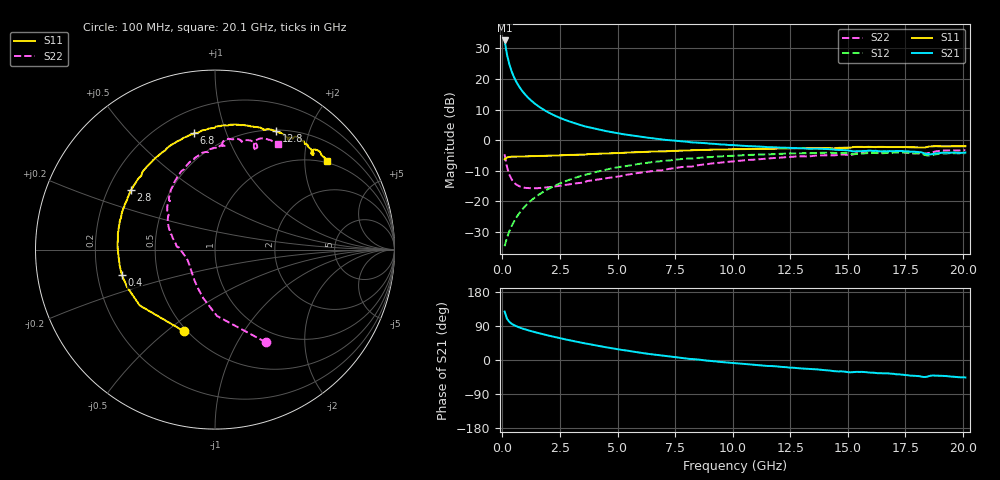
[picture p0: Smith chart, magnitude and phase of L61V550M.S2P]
!  Infineon Technologies AG
! BFR380L3 , PF131585-7, No.6, Th 09.10.01, soldered on pcb-board, measured with PP GSG850
!  Vce=1.5 V,  Ic=50.0 mA
! Common Emitter S-Parameters:  15. November 2001
#  GHz  S  MA  R  50
! f  S11  S21  S12  S22
! GHz  Mag  Ang  Mag  Ang  Mag  Ang  Mag  Ang
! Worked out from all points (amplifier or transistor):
!   201 points, 100 MHz to 20.1 GHz, reference 50 ohm
!   highest |S21| = 32.6 dB at 100 MHz (marker M1)
!   |S21| within 3 dB of that: start of sweep to 166.6 MHz
!   unconditionally stable (mu >= 1): 805.5 MHz to 4.384 GHz; 18.39907 GHz to 18.40202 GHz
!   at 3.4 GHz: K = 1.02, MAG = 7.5 dB, |S12| = -11.7 dB
!   at 10.1 GHz: K = 0.97, MSG = 1.7 dB, |S12| = -5.0 dB
!   at 20.1 GHz: K = 0.99, MSG = 0.1 dB, |S12| = -4.2 dB
!   S11 on the Smith chart (normalised r, x): 100 MHz: 0.48, -0.58; 400 MHz: 0.31, -0.12; 2.8 GHz: 0.30, +0.29; 6.8 GHz: 0.34, +0.78; 12.8 GHz: 0.51, +1.51; 20.1 GHz: 0.95, +2.57
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0.1  0.4871 -110.7  42.69 127.9  0.01857 57.7  0.5886 -61.3
0.2  0.5222 -143.4  25.42 109.3  0.02524 57.5  0.37 -88.3
0.3  0.5323 -157.0  17.69 101.1  0.03225 61.2  0.277 -103.9
0.4  0.538 -164.8  13.49 95.9  0.03929 63.9  0.2309 -115.2
0.5  0.5384 -170.4  10.89 92.2  0.04636 66.2  0.2053 -124.0
0.6  0.5382 -174.4  9.11 89.4  0.05391 67.6  0.1897 -130.7
0.7  0.54 -178.0  7.844 86.8  0.06118 68.7  0.1799 -136.5
0.8  0.5422 179.2  6.883 84.5  0.069 69.3  0.1734 -141.1
0.9  0.5438 176.7  6.134 82.5  0.07656 69.6  0.169 -145.1
1.1  0.5456 172.3  5.049 78.8  0.09205 69.6  0.1654 -151.4
1.4  0.5506 166.4  3.997 73.7  0.115 68.9  0.164 -158.3
1.7  0.5528 161.3  3.316 69.0  0.1378 67.5  0.1665 -163.6
2.2  0.5618 153.4  2.607 61.7  0.175 64.6  0.1746 -170.3
2.8  0.5736 144.8  2.097 53.6  0.2184 60.5  0.1874 -177.2
3.5  0.5817 135.4  1.723 44.8  0.2674 55.4  0.2027 176.4
5.1  0.6174 117.0  1.281 27.3  0.3673 43.1  0.257 160.7
6.8  0.6584 100.3  1.045 12.6  0.4518 30.9  0.3214 143.9
10.1  0.7127 76.2  0.8275 -8.5  0.5607 9.2  0.4545 117.6
12.8  0.7422 62.8  0.7409 -21.5  0.6128 -7.1  0.544 97.5
13.5  0.7447 59.5  0.7286 -24.2  0.6176 -10.9  0.5541 93.4
16.8  0.774 47.5  0.6644 -35.5  0.6207 -26.2  0.6337 74.3
20.1  0.7973 38.3  0.6289 -46.0  0.6142 -39.5  0.6848 59.2
